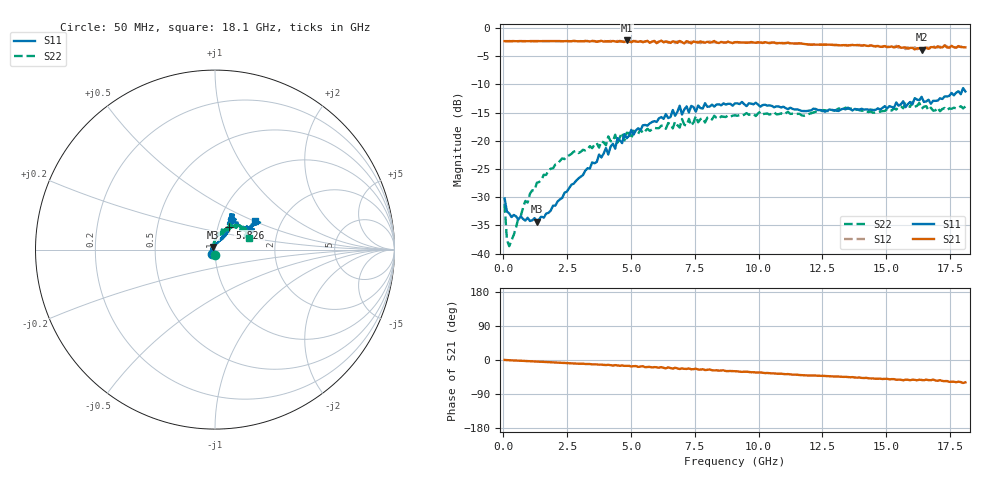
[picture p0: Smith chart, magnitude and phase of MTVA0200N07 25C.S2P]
! Network Analyzer HP8720D.06.14 Serial No. US36140669
! 21 Jun 2005  11:39:35
! Frequency  S11  S21  S12  S22
# HZ  S  DB R 50
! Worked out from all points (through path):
!   201 points, 50 MHz to 18.1 GHz, reference 50 ohm
!   highest |S21| = -2.22 dB at 4.833 GHz (marker M1); lowest = -3.9 dB at 16.39 GHz (marker M2)
!   group delay of S21, straight-line fit = 9.2 ps
!   lowest |S11| = -34.3 dB at 1.313 GHz (marker M3), VSWR 1.04, Z = 48.8 + j1.48 ohm
!   |S11| at or under -10 dB: start of sweep to end of sweep
!   |S22| runs from -38.7 to -13.1 dB; largest |S21 - S12| = 0.039
!   S11 on the Smith chart (normalised r, x): 50 MHz: 0.96, -0.05; 5.826 GHz: 1.13, +0.29; 18.1 GHz: 1.47, +0.50
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5e7  -30.21 -128.2  -2.34 0.1  -2.33 0.1  -31.20 -89.1
1.4025e8  -32.53 -157.3  -2.34 -0.3  -2.35 -0.4  -37.56 -148.0
2.305e8  -32.87 -166.4  -2.35 -0.4  -2.34 -0.7  -38.67 -178.5
8.6225e8  -34.14 147.9  -2.34 -2.6  -2.34 -2.8  -30.66 113.7
1.3135e9  -34.32 127.9  -2.33 -4.1  -2.34 -4.3  -27.44 94.4
3.1185e9  -26.09 65.5  -2.36 -9.7  -2.40 -10.1  -21.59 77.3
4.021e9  -21.28 59.4  -2.37 -13.4  -2.37 -12.7  -20.79 69.0
4.382e9  -21.39 56.9  -2.39 -13.5  -2.40 -14.8  -18.91 68.7
4.47225e9  -19.52 53.4  -2.46 -14.4  -2.30 -13.9  -20.33 72.5
4.83325e9  -19.55 61.4  -2.22 -15.5  -2.41 -16.2  -18.57 61.4
5.826e9  -16.67 57.2  -2.43 -19.7  -2.39 -19.8  -17.98 60.6
6.09675e9  -16.01 57.2  -2.44 -20.3  -2.34 -20.2  -17.75 60.8
6.909e9  -13.78 61.9  -2.31 -23.8  -2.38 -22.3  -17.67 54.7
6.99925e9  -15.35 61.0  -2.53 -22.1  -2.68 -24.1  -16.13 55.5
7.36025e9  -13.82 55.3  -2.73 -24.4  -2.42 -23.8  -17.31 60.8
7.54075e9  -14.84 57.9  -2.49 -22.8  -2.38 -25.7  -15.61 60.7
9.075e9  -13.36 63.8  -2.53 -29.6  -2.50 -30.0  -15.48 52.9
1.21435e10  -14.31 63.4  -2.95 -40.7  -2.90 -41.1  -15.00 48.9
1.512175e10  -13.86 35.4  -3.37 -51.1  -3.19 -51.0  -14.58 37.7
1.638525e10  -12.21 27.8  -3.86 -52.6  -3.54 -52.1  -14.32 26.1
1.674625e10  -13.43 29.3  -3.40 -53.3  -3.64 -54.2  -14.13 22.1
1.81e10  -11.26 35.2  -3.44 -59.0  -3.60 -59.5  -13.92 18.7
